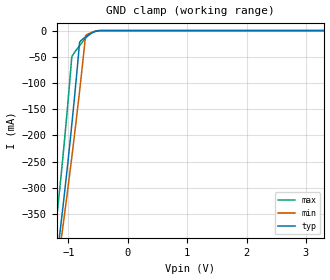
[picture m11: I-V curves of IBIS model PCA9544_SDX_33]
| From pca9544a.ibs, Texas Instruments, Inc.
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[Model]   PCA9544_SDX_33
Model_type  Terminator
| variable   typ   min   max
C_comp   3.12pF   2.52pF   5.65pF
| C_tri-state   3.12pF   2.52pF   5.65pF
[Temperature Range]   40   100   -40
| Ambient temperature   25   85   -40
[Voltage range]   3.3   3   3.6
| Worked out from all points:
|   GND clamp passes 1 mA (typ) near -0.52 V on its own axis
[GND Clamp]
| PCA9544_SDX_33
|   Voltage   I(typ)   I(min)   I(max)
-5.5V     -2.377A    -2.363A    -2.337A
-1.24V    -474.4mA   -493.9mA   -400.8mA
-1.205V   -442.9mA   -466.2mA   -364.9mA
-1.145V   -387.2mA   -417.4mA   -300.6mA
-1.115V   -358.5mA   -392.5mA   -266.9mA
-1.085V   -329.1mA   -367.2mA   -232.1mA
-1.025V   -268.1mA   -315.3mA   -158.8mA
-945mV    -181.8mA   -243.4mA   -52.16mA
-810mV    -21.83mA   -113.4mA   -28.62mA
-710mV    -12.16mA   -9.38mA    -14.54mA
-500mV    -350.2uA   -433uA     -69.41uA
3.3V      117.9pA    368.7pA    75.29pA
